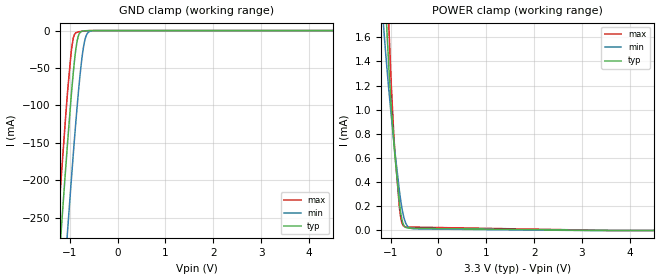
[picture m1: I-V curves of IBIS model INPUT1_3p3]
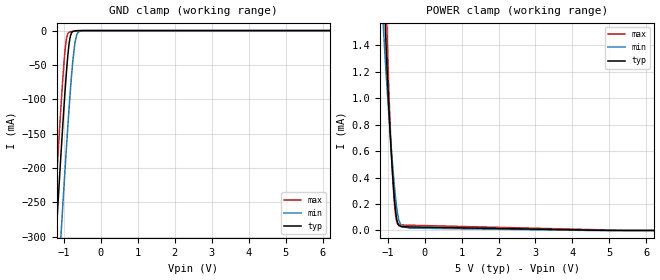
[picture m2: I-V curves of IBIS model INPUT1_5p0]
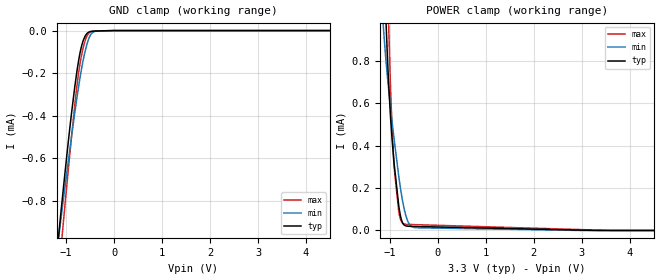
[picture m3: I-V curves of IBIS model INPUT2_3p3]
|Texas Instruments Incorporated
|AMC1035 Delta-Sigma Modulator With Bipolar Input of +/- 1 V and
|Reference Output of 2.5 V
[IBIS Ver]   4.1
[File name]   amc1035.ibs
[Date]   11/30/2018
[File Rev]   1.0
[Source]
| Texas Instruments Incorporated.
| Analog-eLab Design Center, HPA
| 12500 TI Blvd
| Dallas, TX -75243
[Notes]   Revision History:
| Rev 1.0: 11/30/2018
| - Initial version of the model
| - Model generated from simulations in SPECTRE
| - C_comp although listed in numerical order of value are
|   obtained from varying PVT conditions. For PVT conditions for
|   each specific value refer the buffer description under
|   respective [Model]. IBIS model user is responsible for using
|   appropriate C_comp to simulate for Signal Integrity.
| - Warnings regarding combined Non-monotonicity of various models
|   have been reviewed and considered minor and can be ignored.
| - Model names with a trailing _3p3 contain the model for 1.8V operation.
|   Model names with a trailing _5p0 contain the model for 3.3V operation.
[Disclaimer]
| This model is designed as an aid for customers of Texas Instruments.
| TI and its licensors and suppliers make no warranties, either expressed
| or implied, with respect to this  model, including the warranties of
| merchantability or fitness for a particular purpose. The model is
| provided solely on an "as is" basis. The entire risk as to its quality
| and performance is with the customer.
| This model is subject to change without notice. Texas Instruments
| Incorporated is not responsible for updating this model.
[Copyright]
(C) Copyright 2018 Texas Instruments Incorporated.All rights reserved.
|  Component AMC1035D 8 - pin SOIC - D package
|  Part # AMC1035D
[Component]   AMC1035D
[Manufacturer]  TI
[Package]   |8 SOIC - D package
|   typ   min   max
R_pkg   0.05   0.04   0.06
L_pkg   1.0nH   0.8nH   1.2nH
C_pkg   0.2pF   0.16pF   0.24pF
[Pin]   signal_name   model_name   R_pin   L_pin   C_pin
1   MCE   INPUT1   NA   NA   NA
2   AINP   NC   NA   NA   NA
3   AINN   NC   NA   NA   NA
4   REFOUT   NC   NA   NA   NA
5   GND   GND   NA   NA   NA
6   DOUT   OUTPUT   NA   NA   NA
7   CLKIN   INPUT2   NA   NA   NA
8   VDD   POWER   NA   NA   NA
|   Model Selectors
[Model Selector] INPUT1
INPUT1_3p3   3.3V   digital Input
INPUT1_5p0   5.0V   digital Input
[Model Selector] INPUT2
INPUT2_3p3   3.3V   digital Input
INPUT2_5p0   5.0V   digital Input
[Model Selector] OUTPUT
OUTPUT_3p3   3.3V   digital Output
OUTPUT_5p0   5.0V   digital Output
| Models and submodels in the file (6): INPUT1_3p3 (Input), INPUT1_5p0 (Input), INPUT2_3p3 (Input), INPUT2_5p0 (Input), OUTPUT_3p3 (Output), OUTPUT_5p0 (Output)
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|   INPUT1_3p3 Model
[Model]   INPUT1_3p3
Model_type   Input
Vinl = 0.99
Vinh = 2.31
|   typ   min   max
C_comp   5.366E-13   5.031E-13   5.542E-13
|  Where Nom  PVT is Nominal Process, 3.3V,   27C
|   Fast PVT is Strong Process,  3.0V,   -40C
|   Slow PVT is Weak Process,   3.6V,   131C
[Model spec]
|subparameter
Vinl   0.99   0.9   1.08
Vinh   2.31   2.1   2.52
[Voltage Range]   3.3   3   3.6
|Junction Temperature
[Temperature Range]   27   131   -40
[Power Clamp Reference]   3.3   3   3.6
[GND Clamp Reference]   0   0   0
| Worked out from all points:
|   GND clamp passes 1 mA (typ) near -0.75 V on its own axis
|   POWER clamp passes 1 mA (typ) near -0.98 V on its own axis
[GND Clamp]
|   Voltage   I(typ)   I(min)   I(max)
-3.3V     -2.334A    -2.445A    -2.269A
-1.28V    -362.3mA   -482.4mA   -291.2mA
-1.181V   -270.8mA   -390.7mA   -199.8mA
-1.043V   -148mA     -265.6mA   -80.11mA
-953.7mV  -76.26mA   -188.5mA   -20.64mA
-904.2mV  -42.33mA   -147.5mA   -5.787mA
-844.8mV  -13.64mA   -101.3mA   -2.179mA
-765.6mV  -1.603mA   -48.15mA   -1.154mA
-706.2mV  -448.2uA   -19.87mA   -652.2uA
-646.8mV  -154.6uA   -5.58mA    -297.9uA
-557.7mV  -25.7uA    -567.8uA   -51.72uA
6.6V      0A         0A         0A
[POWER Clamp]
|   Voltage   I(typ)   I(min)   I(max)
-3.3V     24.3mA     18.75mA    29.77mA
-1.142V   2.185mA    1.666mA    2.831mA
-1.102V   1.851mA    1.464mA    2.388mA
-1.033V   1.326mA    1.147mA    1.654mA
-983.4mV  1.01mA     939.4uA    1.186mA
-933.9mV  738.5uA    742.7uA    796.6uA
-914.1mV  639.4uA    667.1uA    667.1uA
-815.1mV  225.2uA    325.8uA    188.1uA
-755.7mV  78.64uA    170uA      54.19uA
-676.5mV  24.1uA     54.76uA    29.43uA
-399.3mV  18.39uA    12.49uA    26.87uA
6.6V      0A         0A         0A
|   INPUT1_5p0 Model
[Model]   INPUT1_5p0
Model_type   Input
Vinl = 1.5
Vinh = 3.5
|   typ   min   max
C_comp   5.124E-13   4.849E-13   5.268E-13
|  Where Nom  PVT is Nominal Process,  5.0V,   27C
|   Fast PVT is Strong Process,   5.5V,   -40C
|   Slow PVT is Weak Process,   4.5V,   131C
[Model spec]
|subparameter
Vinl   1.5   1.35   1.65
Vinh   3.5   3.15   3.85
[Voltage Range]   5   4.5   5.5
|Junction Temperature
[Temperature Range]   27   131   -40
[Power Clamp Reference]   5   4.5   5.5
[GND Clamp Reference]   0   0   0
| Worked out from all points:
|   GND clamp passes 1 mA (typ) near -0.74 V on its own axis
|   POWER clamp passes 1 mA (typ) near -0.98 V on its own axis
[GND Clamp]
|   Voltage   I(typ)   I(min)   I(max)
-5V       -4.019A    -4.127A    -3.958A
-1.43V    -503.3mA   -623.1mA   -432.7mA
-1.25V    -334mA     -454.1mA   -262.8mA
-1.16V    -251.4mA   -371.1mA   -180.5mA
-1.085V   -184.4mA   -303.2mA   -114.8mA
-1.04V    -145.6mA   -263.1mA   -77.9mA
-950mV    -73.52mA   -185.4mA   -18.94mA
-845mV    -13.71mA   -101.4mA   -2.183mA
-755mV    -1.235mA   -42.18mA   -1.054mA
-695mV    -365.9uA   -16.1mA    -573.8uA
-500mV    -7.964uA   -130uA     -13.23uA
10V       0A         0A         0A
[POWER Clamp]
|   Voltage   I(typ)   I(min)   I(max)
-5V       42.25mA    32.95mA    51.43mA
-1.115V   1.958mA    1.528mA    2.532mA
-1.055V   1.485mA    1.245mA    1.884mA
-1.025V   1.273mA    1.114mA    1.579mA
-1.01V    1.175mA    1.05mA     1.434mA
-965mV    906.3uA    865.7uA    1.037mA
-920mV    670.9uA    690.2uA    713.2uA
-875mV    461.6uA    524.8uA    458.4uA
-815mV    230.8uA    326.8uA    199.5uA
-740mV    65.48uA    140.3uA    54.56uA
-620mV    28.48uA    29.78uA    41.16uA
10V       0A         0A         0A
|   INPUT2_3p3 Model
[Model]   INPUT2_3p3
Model_type   Input
Vinl = 0.99
Vinh = 2.31
|   typ   min   max
C_comp   2.580E-13   2.509E-13   2.652E-13
|  Where Nom  PVT is Nominal Process, 3.3V,   27C
|   Fast PVT is Strong Process,  3.6V,   -40C
|   Slow PVT is Weak Process,   3.0V,   131C
[Model spec]
|subparameter
Vinl   0.99   0.9   1.08
Vinh   2.31   2.1   2.52
[Voltage Range]   3.3   3   3.6
|Junction Temperature
[Temperature Range]   27   131   -40
[Power Clamp Reference]   3.3   3   3.6
[GND Clamp Reference]   0   0   0
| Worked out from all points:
|   GND clamp passes 1 mA (typ) near -1.17 V on its own axis
|   POWER clamp passes 1 mA (typ) near -1.08 V on its own axis
[GND Clamp]
|   Voltage   I(typ)   I(min)   I(max)
-3.3V     -6.124mA   -5.016mA   -7.439mA
-1.221V   -1.11mA    -1.089mA   -1.307mA
-1.102V   -840.7uA   -874.1uA   -1.011mA
-1.092V   -818.7uA   -856.3uA   -986.3uA
-1.053V   -731.4uA   -785.7uA   -889.5uA
-884.4mV  -382.5uA   -493.5uA   -492uA
-745.8mV  -149.4uA   -272.4uA   -208.5uA
-636.9mV  -42.91uA   -131.3uA   -74.16uA
-508.2mV  -5.46uA    -27.75uA   -8.817uA
-409.2mV  -2.237uA   -4.156uA   -2.981uA
-122.1mV  -604.9nA   -444.8nA   -819.5nA
6.6V      0A         0A         0A
[POWER Clamp]
|   Voltage   I(typ)   I(min)   I(max)
-3.3V     20.66mA    15.37mA    26.17mA
-1.142V   1.378mA    978.7uA    2.033mA
-1.092V   1.052mA    829.7uA    1.557mA
-1.053V   826.4uA    728.5uA    1.199mA
-1.023V   682.3uA    659.6uA    949.8uA
-953.7mV  429.1uA    512.9uA    478.2uA
-914.1mV  321.3uA    434.8uA    303.9uA
-805.2mV  102uA      240uA      77.32uA
-676.5mV  22.53uA    78.02uA    29.58uA
-587.4mV  19.6uA     27.01uA    28.32uA
-399.3mV  18.49uA    12.62uA    27.01uA
6.6V      0A         0A         0A
